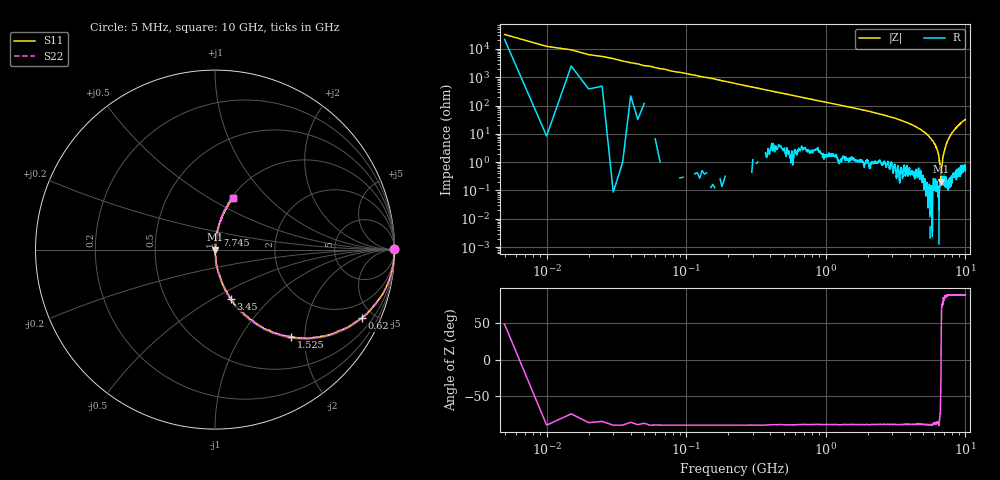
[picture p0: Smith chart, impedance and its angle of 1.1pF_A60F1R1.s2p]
! Amotech Co.,Ltd.
! http://www.amotech.co.kr/
! Part Number: A60F1R1
! These Parameters are Measured in Series Mode Connection
! Operation Temp=25[degC], DC Bias Voltage=0[V]
! Freq. Start=5[MHz] Stop=10[GHz], 2000[Steps]
! Date: Monday, July 20, 2020, 03:50:51
# GHZ S RI R 50.000000
!Freq.(Hz) S11(Real) S11(Imag) S21(Real) S21(Imag) S12(Real) S12(Imag) S22(Real) S22(Imag)
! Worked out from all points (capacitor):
!   2000 points, 5 MHz to 10 GHz, reference 50 ohm
!   read as one part in series: C = 1.19 pF near 55 MHz
!   lowest |Z| = 203 mohm at 6.695 GHz (marker M1)
!   series resonance near 6.694 GHz, so ESL is about 480 pH
!   S11 on the Smith chart (normalised r, x): 5 MHz: open; 620 MHz: 1.04, -4.27; 1.525 GHz: 1.03, -1.70; 3.45 GHz: 1.01, -0.60; 7.745 GHz: 1.01, +0.16; 10 GHz: 1.01, +0.65
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0.005  0.998 0.0023  0.00205 -0.0023  0.00205 -0.0023  0.998 0.0023
0.07  0.9973 -0.0516  0.00266 0.0516  0.00266 0.0516  0.9973 -0.0516
0.155  0.9877 -0.1101  0.0123 0.1101  0.0123 0.1101  0.9877 -0.1101
0.33  0.9424 -0.2333  0.0576 0.2333  0.0576 0.2333  0.9424 -0.2333
0.62  0.8181 -0.3816  0.1819 0.3816  0.1819 0.3816  0.8181 -0.3816
1.525  0.4222 -0.4855  0.5778 0.4855  0.5778 0.4855  0.4222 -0.4855
1.675  0.3765 -0.4777  0.6235 0.4777  0.6235 0.4777  0.3765 -0.4777
3.34  0.0939 -0.2859  0.9061 0.2859  0.9061 0.2859  0.0939 -0.2859
3.45  0.0884 -0.2732  0.9116 0.2732  0.9116 0.2732  0.0884 -0.2732
5.005  0.016 -0.1183  0.984 0.1183  0.984 0.1183  0.016 -0.1183
5.84  0.00418 -0.0569  0.9958 0.0569  0.9958 0.0569  0.00418 -0.0569
6.285  0.00243 -0.0271  0.9976 0.0271  0.9976 0.0271  0.00243 -0.0271
6.48  0.000571 -0.0134  0.9994 0.0134  0.9994 0.0134  0.000571 -0.0134
6.57  0.00149 -0.0077  0.9985 0.0077  0.9985 0.0077  0.00149 -0.0077
6.67  0.002 -0.00134  0.998 0.00134  0.998 0.00134  0.002 -0.00134
6.695  0.00203 8.25e-05  0.998 -8.25e-05  0.998 -8.25e-05  0.00203 8.25e-05
6.87  0.00301 0.0119  0.997 -0.0119  0.997 -0.0119  0.00301 0.0119
6.96  0.00185 0.0177  0.9981 -0.0177  0.9981 -0.0177  0.00185 0.0177
7.295  0.00364 0.0442  0.9964 -0.0442  0.9964 -0.0442  0.00364 0.0442
7.745  0.00921 0.0808  0.9908 -0.0808  0.9908 -0.0808  0.00921 0.0808
8.335  0.0228 0.1352  0.9772 -0.1352  0.9772 -0.1352  0.0228 0.1352
10  0.0994 0.2893  0.9006 -0.2893  0.9006 -0.2893  0.0994 0.2893
